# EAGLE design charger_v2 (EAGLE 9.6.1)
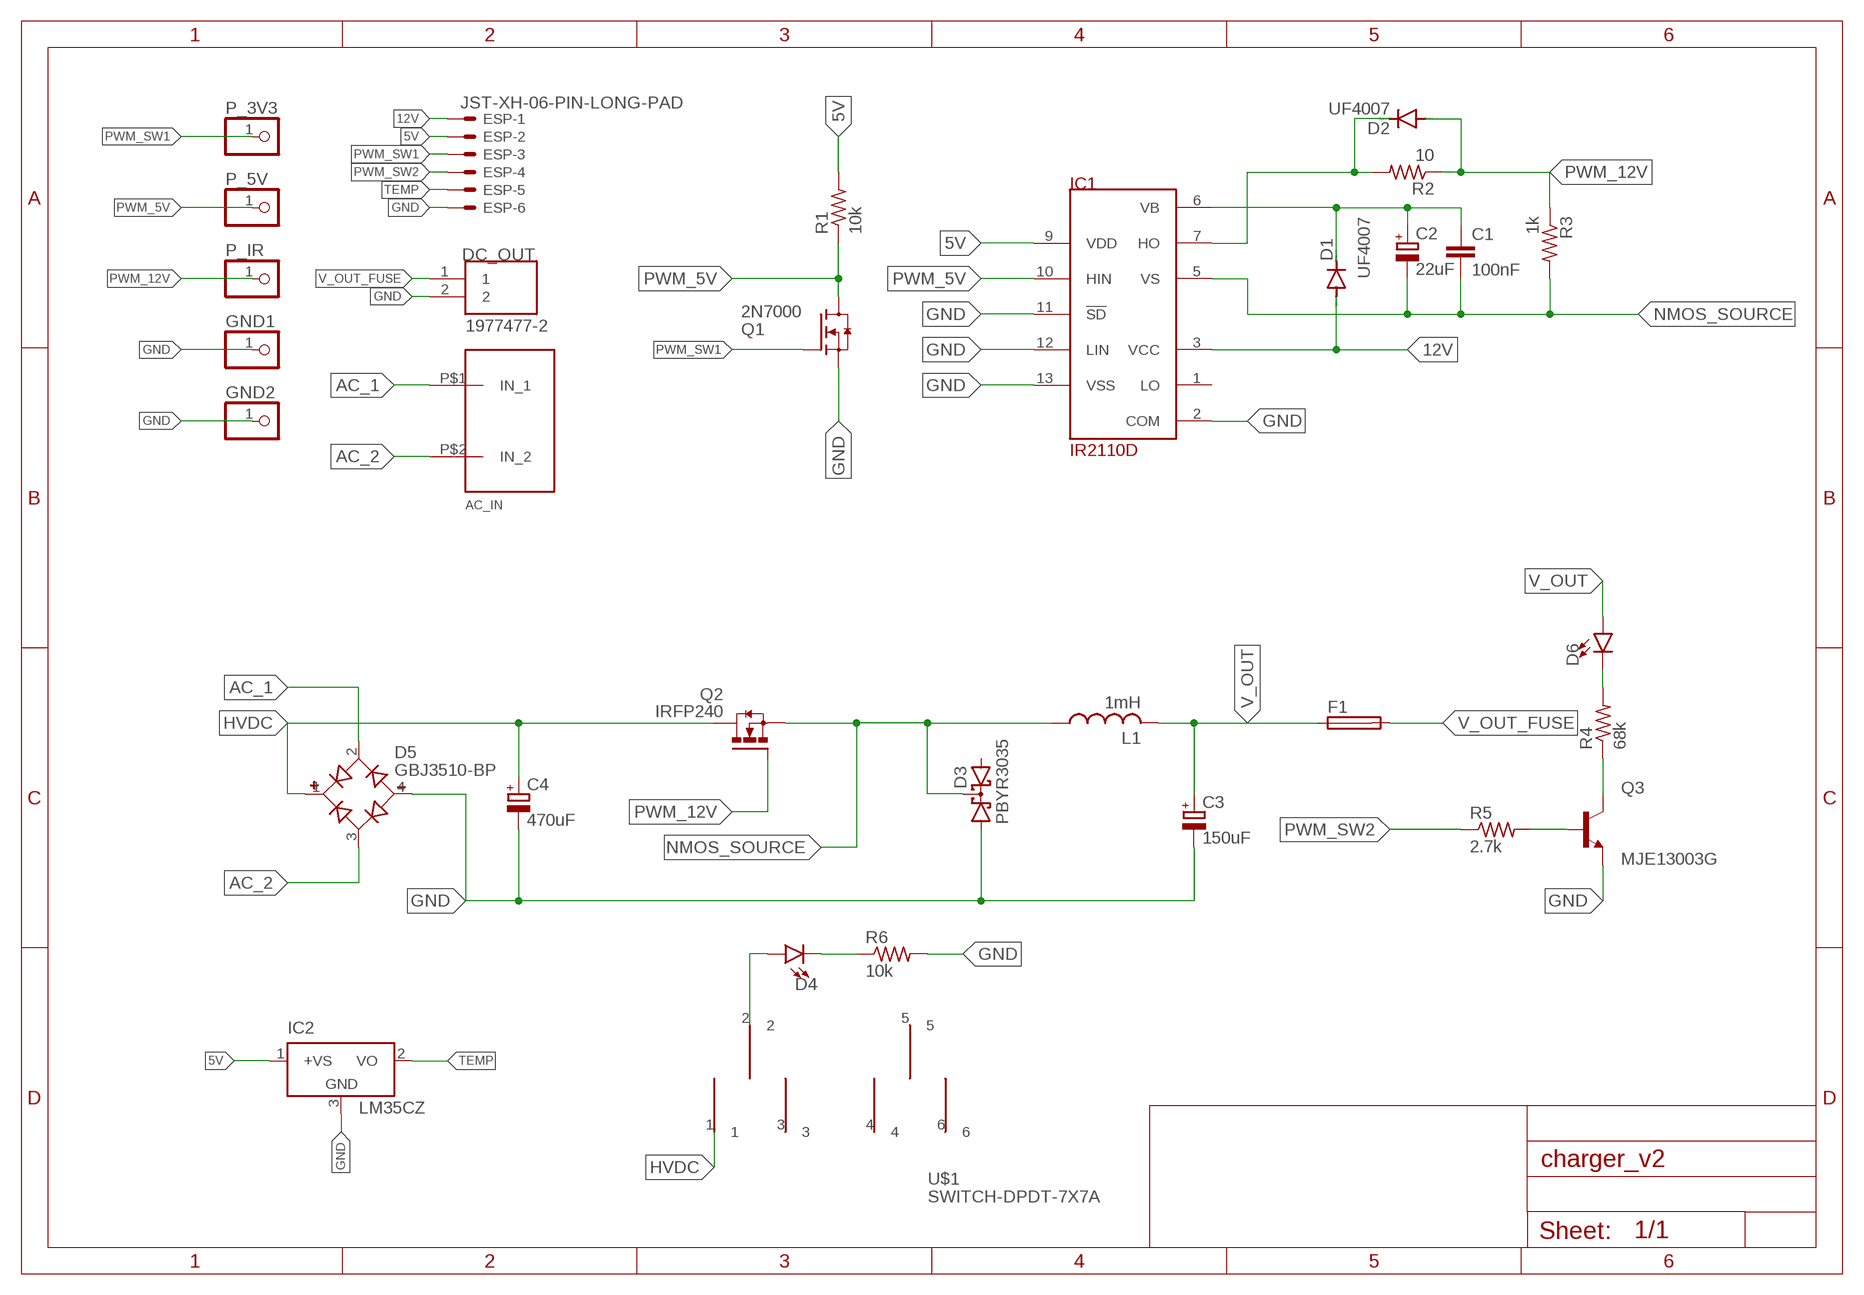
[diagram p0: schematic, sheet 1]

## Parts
AC_IN  XT90A  [XT90-PAD]
C1  100nF  C-EU025-025X050  [C025-025X050]
C2  22uF  CPOL-EUE2,5-6E  [E2,5-6E]
C3  150uF  CPOL-EUE7.5-18  [E7,5-18]
C4  470uF  CPOL-EUE10-35  [EB35D]
D1  UF4007  BAS15  [DO34-7]
D2  UF4007  BAS15  [DO34-7]
D3  PBYR3035  [SOT93S]
D4  LED5MM  [LED_5MM]
D5  GBJ3510-BP  [DIOB_GBJ3510-BP]
D6  LED5MM  [LED_5MM]
DC_OUT  1977477-2  [TE_1977477-2]
ESP  JST-XH-06-PIN-LONG-PAD  [JST-XH-06-PACKAGE-LONG-PAD]
F1  SH25  [SH25]
GND1  PINHD-1X1  [1X01]
GND2  PINHD-1X1  [1X01]
IC1  IR2110D  [DIL14]
IC2  LM35CZ  [TO92]
L1  1mH  L-USTJ7-U1  [TJ7-U1]
P_3V3  PINHD-1X1  [1X01]
P_5V  PINHD-1X1  [1X01]
P_IR  PINHD-1X1  [1X01]
Q1  2N7000  [TO92]
Q2  IRFP240  [TO247AC]
Q3  MJE13003G  [TO229P780X300X1364-3]
R1  10k  R-US_0204/7  [0204/7]
R2  10  R-US_0204/7  [0204/7]
R3  1k  R-US_0204/7  [0204/7]
R4  68k  R-US_0309/12  [0309/12]
R5  2.7k  R-US_0204/7  [0204/7]
R6  10k  R-US_0204/7  [0204/7]
U$1  SWITCH-DPDT-7X7A  [TL-2230]

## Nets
5V: ESP.2 IC1.9(VDD) IC2.1(+VS) R1.2
12V: D1.A ESP.1 IC1.3(VCC)
AC_1 [power]: AC_IN.P$1(IN_1) D5.2(AC1)
AC_2 [power]: AC_IN.P$2(IN_2) D5.3(AC2)
GND: C3.- C4.- D3.A1 D5.4(-) DC_OUT.2 ESP.6 GND1.1 GND2.1 IC1.2(COM) IC1.11(!SD) IC1.12(LIN) IC1.13(VSS) IC2.3(GND) Q1.1(S) Q3.3(E) R6.2
HVDC [power]: C4.+ D5.1(+) Q2.2(D) U$1.1
N$1: D2.C IC1.7(HO) R2.2
N$2: D4.A U$1.2
N$3: Q3.2(C) R4.1
N$4: D6.K(C) R4.2
N$5: Q3.1(B) R5.2
N$8: D4.K(C) R6.1
NMOS_SOURCE [power]: C1.2 C2.- D3.C IC1.5(VS) L1.1 Q2.3(S) R3.2
PWM_5V: IC1.10(HIN) P_5V.1 Q1.3(D) R1.1
PWM_12V [pwm_12]: D2.A P_IR.1 Q2.1(G) R2.1 R3.1
PWM_SW1: ESP.3 P_3V3.1 Q1.2(G)
PWM_SW2: ESP.4 R5.1
TEMP: ESP.5 IC2.2(VO)
V_OUT [power]: C3.+ D6.A F1.1 L1.2
V_OUT_FUSE [power]: DC_OUT.1 F1.2
VB: C1.1 C2.+ D1.C IC1.6(VB)
Unconnected: D3.A2 IC1.1(LO) U$1.3 U$1.4 U$1.5 U$1.6

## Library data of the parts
AC_IN = TA_library:XT90
C1 = rcl:C-EU: CAPACITOR, European symbol; SPICEPREFIX: C
C2-C4 = rcl:CPOL-EU: POLARIZED CAPACITOR, European symbol; SPICEPREFIX: C
D1 D2 = diode:BAS15: DIODE
D3 = diode:PBYR3035: Dual DIODE common cathode
D4 D6 = Sparkfun_LED:LED: LED (Generic)
D5 = GBJ3510-BP:GBJ3510-BP: Diode Rectifier Bridge Single 1KV 35A 4-Pin(4+Tab) Case GBJ Bulk/Tube Check availability; AVAILABILITY: In Stock; DESCRIPTION: Bridge Rectifier Single Phase Standard 1 kV Through Hole GBJ; MF: Micro Commercial; MP: GBJ3510-BP; PACKAGE: SIP-4 Micro Commercial Co; PRICE: None; PURCHASE-URL: https://pricing.snapeda.com/search/part/GBJ3510-BP/?ref=eda
DC_OUT = terminal_block_TA:1977477-2: Check availability; AVAILABILITY: In Stock; COMMENT: 1977477-2; DESCRIPTION: Conn Barrier Strip 2 POS 8.25mm Solder ST Thru-Hole 15A/Contact Carton; MF: TE Connectivity; MP: 1977477-2; PACKAGE: None; PRICE: None; PURCHASE-URL: https://pricing.snapeda.com/search/part/1977477-2/?ref=eda
ESP = Rembrandt Electronics - JST XH Connectors v1-0:JST-XH-06-PIN: JST XH Connector 2 Pin Wire to board connector. Pitch: 2,54 mm, (0.100") Number of pins: 6 Created by Rembrandt Electronics www.rembrandtelectronics.com
F1 = fuse:SH25: FUSE HOLDER; MF: SCHURTER; MPN: 0031.8211; OC_FARNELL: 1162741; OC_NEWARK: 96B9380
GND1 GND2 P_3V3 P_5V P_IR = pinhead:PINHD-1X1: PIN HEADER
IC1 = irs:IR2110
IC2 = lm35:LM35: Single-Supply Centigrade Temperature Sensor Vout = (10mV/°C x Temp °C) +5mmmV Source: http://www.national.com/ds/LM/LM35.pdf
L1 = custom_inductor:L-US: INDUCTOR, American symbol; SPICEPREFIX: L
Q1 = 2N7000:2N7000: Check prices; AVAILABILITY: In Stock; DESCRIPTION: N-Channel 60V 350mA (Tc) 1W (Tc) Through Hole TO-92-3; MF: STMicroelectronics; MP: 2N7000; PACKAGE: E-PKG AXIAL-LEADED-2 ON Semiconductor; PRICE: None
Q2 = IRFP240(TO-247):IRFP240: MOSFET N-CH 200V 20A TO-247AC Check availability; AVAILABILITY: In Stock; DESCRIPTION: N-Channel 200 V 20A (Tc) 150W (Tc) Through Hole TO-247AC; MF: Vishay Siliconix; MP: IRFP240; PACKAGE: TO-247 Vishay Siliconix; PRICE: None
Q3 = MJE13003G:MJE13003G: Bipolar (BJT) Transistor NPN 400V 1.5A 10MHz 1.4W Through Hole TO-225AA Check availability; AVAILABILITY: Not in stock; DESCRIPTION: Bipolar (BJT) Transistor NPN 400 V 1.5 A 10MHz 1.4 W Through Hole TO-126; MF: ON Semiconductor; MP: MJE13003G; PACKAGE: TO-126 ON Semiconductor; PRICE: None
R1-R6 = rcl:R-US_: RESISTOR, American symbol; SPICEPREFIX: R
U$1 = TA_library:SWITCH-DPDT-7X7

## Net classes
0 default: width 0.305 mm
1 power: width 6.985 mm, clearance 0.508 mm to class 0
2 pwm_12: width 0.305 mm, clearance 0.508 mm to class 0, clearance 0.508 mm to class 1

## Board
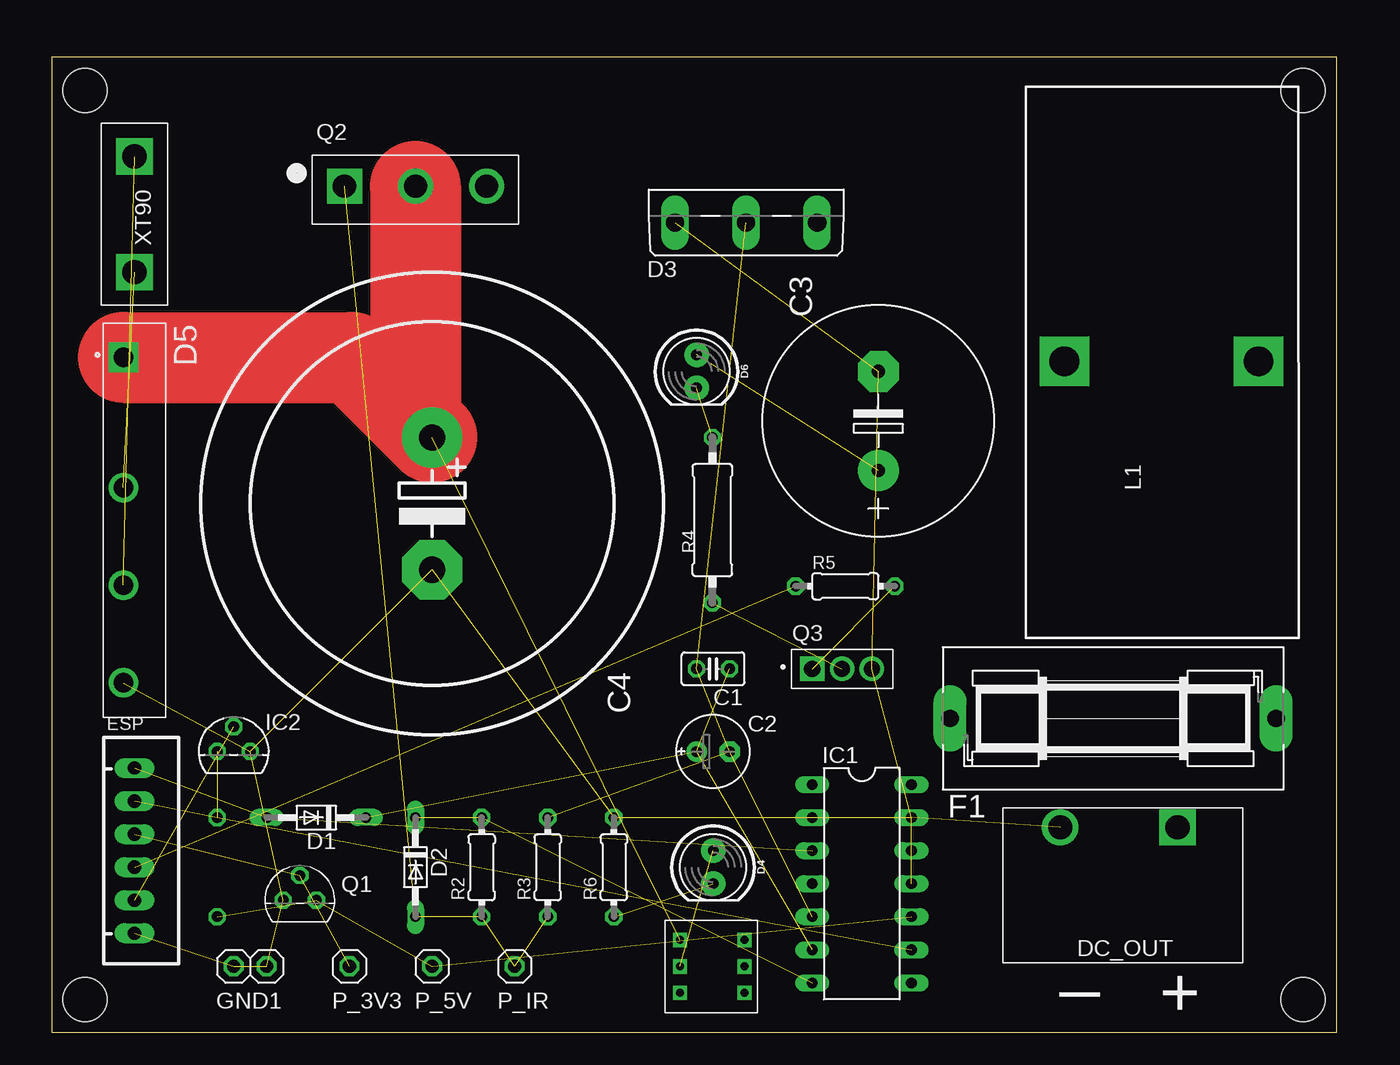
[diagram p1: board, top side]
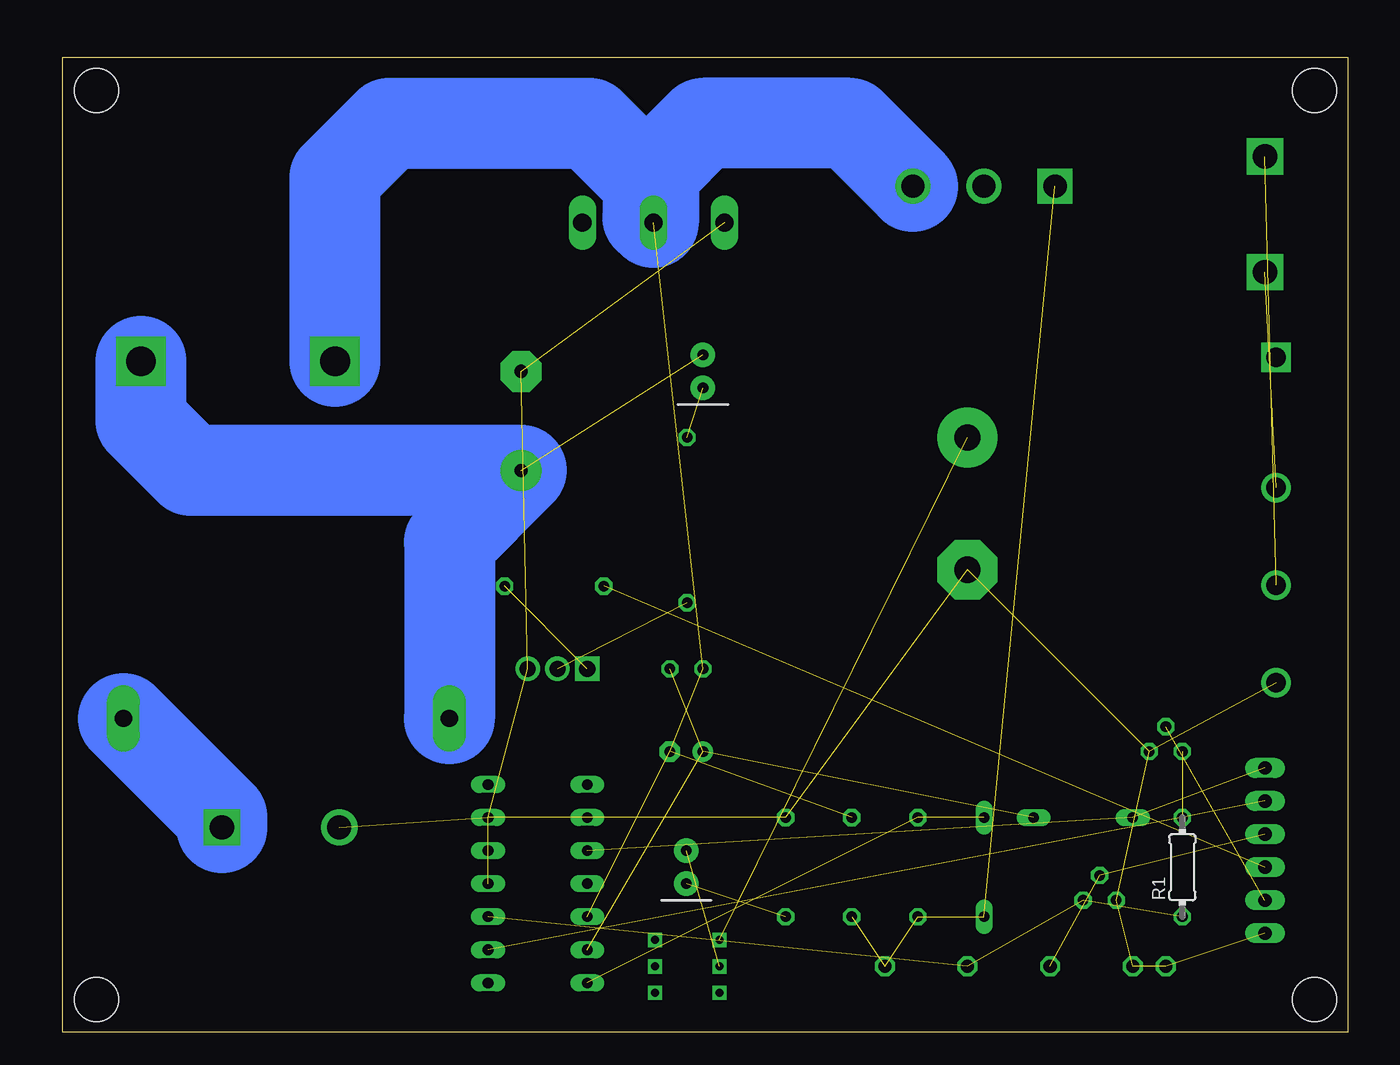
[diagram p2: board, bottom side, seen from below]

Size 98.73 x 74.92 mm. Coordinates in mm from the lower left corner, seen from the top.
Outline: 0,0 98.73,0 98.73,74.92 0,74.92 0,0
Copper layers (1*16): Top 0.035mm / dielectric 1.5mm / Bottom 0.035mm
Design rules "default *": minimum track width 12mil, minimum drill 0.35mm, track to track 12mil, track to pad 12mil, pad to pad 12mil, via to via 12mil, smd to smd 12mil, copper to edge 40mil, drill to drill 6mil, minimum pad ring 10mil, minimum via ring 8mil, stop-mask expansion 4mil, vias tented up to drill 0mil, thermal gap 10mil
Holes 3.4 mm at 2.54,72.39 96.14,72.39 2.54,2.54 96.14,2.54

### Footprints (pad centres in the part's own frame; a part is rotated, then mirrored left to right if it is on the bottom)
XT90-PAD = drill 1.854 square: P$1 0,5.08; P$2 0,-3.81
C025-025X050 = drill 0.813 octagon: 1 -1.27,0; 2 1.27,0
E2,5-6E = drill 0.813 pad 1.575: + -1.27,0 | drill 0.813 pad 1.575 octagon: - 1.27,0
E7,5-18 = drill 1.016 pad 3.15: + -3.81,0 | drill 1.016 pad 3.15 octagon: - 3.81,0
EB35D = drill 2.007 pad 4.597: + -5.08,0 | drill 2.007 pad 4.597 octagon: - 5.08,0
DO34-7 = drill 0.813 long: A 3.81,0; C -3.81,0
SOT93S = drill 1.397 long: A1 -5.461,-2.54; A2 5.461,-2.54; C 0,-2.54
LED_5MM = drill 0.813 pad 1.88: A -1.27,0; K 1.27,0
DIOB_GBJ3510-BP = drill 1.51 pad 2.27 square: 1 -12.5,-0.85 | drill 1.51 pad 2.27: 2 -2.5,-0.85; 3 5,-0.85; 4 12.5,-0.85
TE_1977477-2 = drill 1.85 square: 1 -3.241,-5.334 | drill 1.85: 2 5.781,-5.334
JST-XH-06-PACKAGE-LONG-PAD = drill 1.016 long: 1 -6.35,0; 2 -3.81,0; 3 -1.27,0; 4 1.27,0; 5 3.81,0; 6 6.35,0
SH25 = drill 1.321 pad 2.54 long: 1 -12.522,0; 2 12.522,0
1X01 = drill 1.016 octagon: 1 0,0
DIL14 = drill 0.813 long: 1 -7.62,-3.81; 2 -5.08,-3.81; 3 -2.54,-3.81; 4 0,-3.81; 5 2.54,-3.81; 6 5.08,-3.81; 7 7.62,-3.81; 8 7.62,3.81; 9 5.08,3.81; 10 2.54,3.81; 11 0,3.81; 12 -2.54,3.81; 13 -5.08,3.81; 14 -7.62,3.81
TO92 = drill 0.813 octagon: 1 -1.27,0; 2 0,1.905; 3 1.27,0
TJ7-U1 = drill 2.286 pad 3.81 square: 1 -6.503,4.826; 2 8.408,4.826
TO247AC = drill 1.79 pad 2.69 square: 1 -5.46,0.255 | drill 1.79 pad 2.69: 2 0,0.255; 3 5.46,0.255
TO229P780X300X1364-3 = drill 1.25 square: 1 0,0 | drill 1.25: 2 2.29,0; 3 4.58,0
0204/7 = drill 0.813 octagon: 1 -3.81,0; 2 3.81,0
0309/12 = drill 0.813 octagon: 1 -6.35,0; 2 6.35,0
TL-2230 = drill 0.6 square: 1 -2.032,-2.54; 2 0,-2.54; 3 2.032,-2.54; 4 -2.032,2.413; 5 0,2.413; 6 2.032,2.413

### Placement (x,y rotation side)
AC_IN  6.35,63.5 180 top
C1  50.8,27.94 180 top
C2  50.8,21.59 0 top
C3  63.5,46.99 90 top
C4  29.21,40.64 270 top
D1  20.32,16.51 180 top
D2  27.94,12.7 270 top
D3  53.34,64.77 0 top
D4  50.8,12.7 270 top
D5  6.35,39.37 270 top
D6  49.53,50.8 270 top
DC_OUT  83.25,10.41 180 top
ESP  6.35,13.97 270 top
F1  81.53,24.13 0 top
GND1  13.97,5.08 0 top
GND2  16.51,5.08 0 top
IC1  62.23,11.43 270 top
IC2  13.97,21.59 0 top
L1  84.3,46.74 0 top
P_3V3  22.86,5.08 0 top
P_5V  29.21,5.08 0 top
P_IR  35.56,5.08 0 top
Q1  19.05,10.16 0 top
Q2  27.94,64.77 0 top
Q3  58.42,27.94 0 top
R1  12.7,12.7 90 bottom
R2  33.02,12.7 90 top
R3  38.1,12.7 90 top
R4  50.75,39.37 90 top
R5  60.96,34.29 0 top
R6  43.18,12.7 90 top
U$1  50.8,5.08 270 top

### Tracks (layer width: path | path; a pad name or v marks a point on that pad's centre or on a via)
5V  (3 unrouted)
12V  (2 unrouted)
AC_1  (1 unrouted)
AC_2  (1 unrouted)
GND  (15 unrouted)
HVDC  (1 unrouted)
  Top 6.985: D5.1 23.06,51.87 C4.+ 27.94,46.99 Q2.2
N$1  (2 unrouted)
N$2  (1 unrouted)
N$3  (1 unrouted)
N$4  (1 unrouted)
N$5  (1 unrouted)
N$8  (1 unrouted)
NMOS_SOURCE  (4 unrouted)
  Bottom 6.985: Q2.3 38.23,69.85 49.53,69.85 53.34,66.04 D3.C 53.75,62.64 53.75,65.37 58.23,69.85 73.66,69.85 77.8,65.71 L1.1
PWM_5V  (3 unrouted)
PWM_12V  (4 unrouted)
PWM_SW1  (2 unrouted)
PWM_SW2  (1 unrouted)
TEMP  (1 unrouted)
V_OUT  (1 unrouted)
  Bottom 6.985: L1.2 92.71,46.99 88.9,43.18 C3.+ 69.01,37.67 F1.1
V_OUT_FUSE
  Bottom 6.985: F1.2 86.49,16.57 DC_OUT.1
VB  (3 unrouted)

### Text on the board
tPlace: _ | +

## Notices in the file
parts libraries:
Sparkfun_LED: Licensing: Creative Commons ShareAlike 4.0 International - https://creativecommons.org/licenses/by-sa/4.0
